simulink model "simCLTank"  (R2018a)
settings: Solver=ode15s  StartTime=0.0  StopTime=tsim  RelTol=1e-3
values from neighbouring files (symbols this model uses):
  dnom = zeros(2,1)    [PI_Tank.m]    (also in runCascade.m)
  dstep = dnom + dnom.*[0;0]    [PI_Tank.m]
  Kc = 0    [PI_Tank.m]    (also in runCascade.m = tauQ/(tauC+theta); runTransformedMVs.m = 0.01; Main.m = 1/k*tau/(tauC+theta); runTransf.m = 1/kM(i)*tau(i)/(tauCM(i)+theta(i)))
  p = [V;rho;cp;qnom;MV;transf]    [PI_Tank.m]    (also in runCascade.m = [V;rho;cp;A;tau0;MV;transf]; runTransformedMVs.m = [V;rho;cp;A;tau0;MV;transf]; Main.m = [N, Fc0, rhoc, rhoh,U,A,cpc,cph]; Main_OL.m = [N, Fc0, rhoc, rhoh,U,A,cpc,cph])
  tauI = 1    [PI_Tank.m]    (also in runCascade.m = min(tauQ,4*(tauC+theta)); runTransformedMVs.m = 400; Main.m = min(tau,4*(tauC+theta)); runTransf.m = min(tau(i), 4*(tauCM(i)+theta(i))))
  Tnom = 50    [PI_Tank.m]    (also in runCascade.m; runTransformedMVs.m)
  Tstep = Tnom+10    (= 60)    [PI_Tank.m]    (also in runCascade.m = 40; runTransformedMVs.m = -10)
  tstep_d = 10    [PI_Tank.m]    (also in runCascade.m)
  tstep_T = 50    [PI_Tank.m]    (also in runCascade.m = 500)
  ubias = Qnom    (= 167.2)    [PI_Tank.m]    (also in runCascade.m = 1672; runTransformedMVs.m = 1672)
undefined symbols (not defined in the file or in its folder): Tank

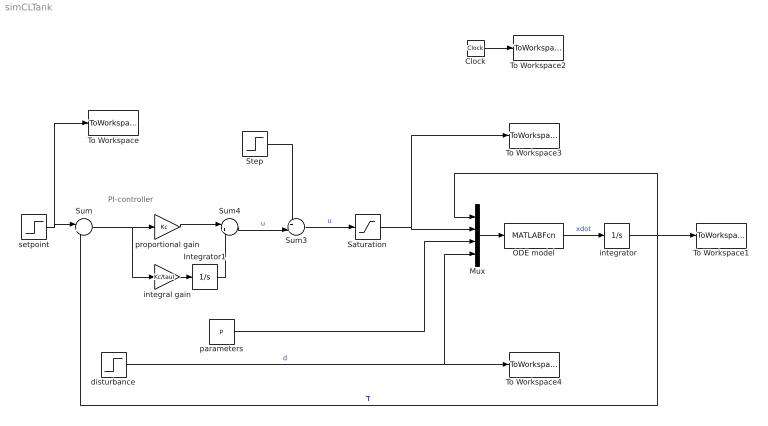
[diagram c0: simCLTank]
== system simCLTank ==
  note: PI-controller
  " integrator" : Integrator  InitialCondition=Tnom
  Clock : Clock
  Integrator1 : Integrator
  Mux : Mux
  ODE model : MATLABFcn  MATLABFcn=Tank(u(1), u(2),u(3:8),u(9:10))  OutputDimensions=1
  Saturation : Saturate  UpperLimit=inf  LowerLimit=-inf
  Step : Step  Time=50  Before=ubias  After=ubias*1.1  SampleTime=0
  Sum : Sum  Inputs=|+-
  Sum3 : Sum  Inputs=++|
  Sum4 : Sum  Inputs=|++
  To Workspace : ToWorkspace  VariableName=Tsp  SampleTime=-1
  To Workspace1 : ToWorkspace  VariableName=T  SampleTime=-1
  To Workspace2 : ToWorkspace  VariableName=time  SampleTime=-1
  To Workspace3 : ToWorkspace  VariableName=u  SampleTime=-1
  To Workspace4 : ToWorkspace  VariableName=d  SampleTime=-1
  disturbance : Step  Time=tstep_d  Before=dnom  After=dstep  SampleTime=0
  integral gain : Gain  Gain=Kc/tauI  Multiplication=Matrix(K*u)
  parameters : Constant  Value=p
  proportional gain : Gain  Gain=Kc  Multiplication=Matrix(K*u)
  setpoint : Step  Time=tstep_T  Before=Tnom  After=Tstep  SampleTime=0
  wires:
  " integrator"/1 -> Mux/1, Sum/2, To Workspace1/1  "T"
  Mux/1 -> ODE model/1
  Clock/1 -> To Workspace2/1
  Sum/1 -> integral gain/1, proportional gain/1
  Sum3/1 -> Saturation/1  "u"
  Sum4/1 -> Sum3/2  "u"
  ODE model/1 -> " integrator"/1  "xdot"
  integral gain/1 -> Integrator1/1
  proportional gain/1 -> Sum4/1
  Integrator1/1 -> Sum4/2
  disturbance/1 -> Mux/4, To Workspace4/1  "d"
  parameters/1 -> Mux/3
  Step/1 -> Sum3/1
  setpoint/1 -> To Workspace/1, Sum/1
  Saturation/1 -> Mux/2, To Workspace3/1
